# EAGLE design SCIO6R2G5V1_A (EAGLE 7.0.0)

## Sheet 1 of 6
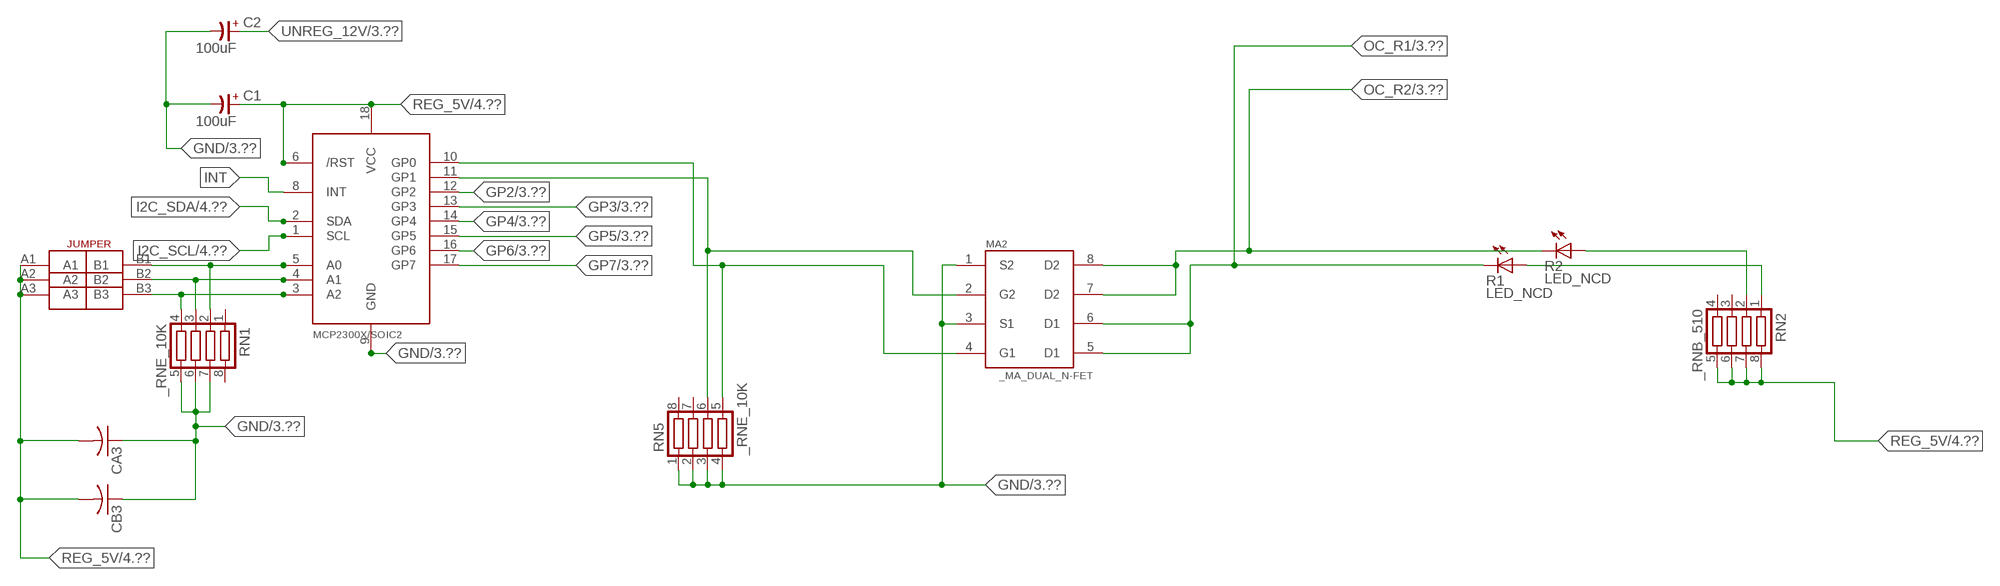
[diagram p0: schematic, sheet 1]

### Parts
C1  100uF  CP-E-025X060  [E-025X060]
C2  100uF  CP-E-025X060  [E-025X060]
CA3  CC1206KRX7R9BB104C1206K  [CC1206KRX7R9BB104]
CB3  TMK316F106ZL-TC1206K  [TMK316F106ZL-T]
IC2  MCP2300X/SO  [SO18W]
MA2  _MA_DUAL_N-FET  [_MA_DUAL_N-FET]
R1  LED_NCD  [CHIPLED_0603]
R2  LED_NCD  [CHIPLED_0603]
RN1  _RNE_10K  [RNE]
RN2  _RNB_510  [RNB]
RN5  _RNE_10K  [RNE]
U$18  JUMPER_3X2  [JUMPER_3X2]

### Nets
GND: C1.- C2.- CA3.1 CB3.1 IC2.9(GND) MA2.1(S2) MA2.3(S1) RN1.5 RN1.6 RN1.7 RN5.1 RN5.2 RN5.3 RN5.4 ; also sheet 3,4,6
GP2: IC2.12(GP2) ; also sheet 3
GP3: IC2.13(GP3) ; also sheet 3
GP4: IC2.14(GP4) ; also sheet 3
GP5: IC2.15(GP5) ; also sheet 3
GP6: IC2.16(GP6) ; also sheet 3
GP7: IC2.17(GP7) ; also sheet 3
I2C_SCL: IC2.1(SCL) ; also sheet 4
I2C_SDA: IC2.2(SDA) ; also sheet 4
INT: IC2.8(INT)
N$6: IC2.5(A0) RN1.2 U$18.B1
N$7: IC2.4(A1) RN1.3 U$18.B2
N$8: IC2.3(A2) RN1.4 U$18.B3
N$22: IC2.11(GP1) MA2.2(G2) RN5.6
N$23: IC2.10(GP0) MA2.4(G1) RN5.5
N$31: R2.A RN2.2
N$32: R1.A RN2.1
OC_R1: MA2.5(D1) MA2.6(D1) R1.C ; also sheet 3
OC_R2: MA2.7(D2) MA2.8(D2) R2.C ; also sheet 3
REG_5V: C1.+ CA3.2 CB3.2 IC2.6(/RST) IC2.18(VCC) RN2.5 RN2.6 RN2.7 RN2.8 U$18.A1 U$18.A2 U$18.A3 ; also sheet 4,6
UNREG_12V: C2.+ ; also sheet 3,4
Unconnected: RN1.1 RN1.8 RN2.3 RN2.4 RN5.7 RN5.8

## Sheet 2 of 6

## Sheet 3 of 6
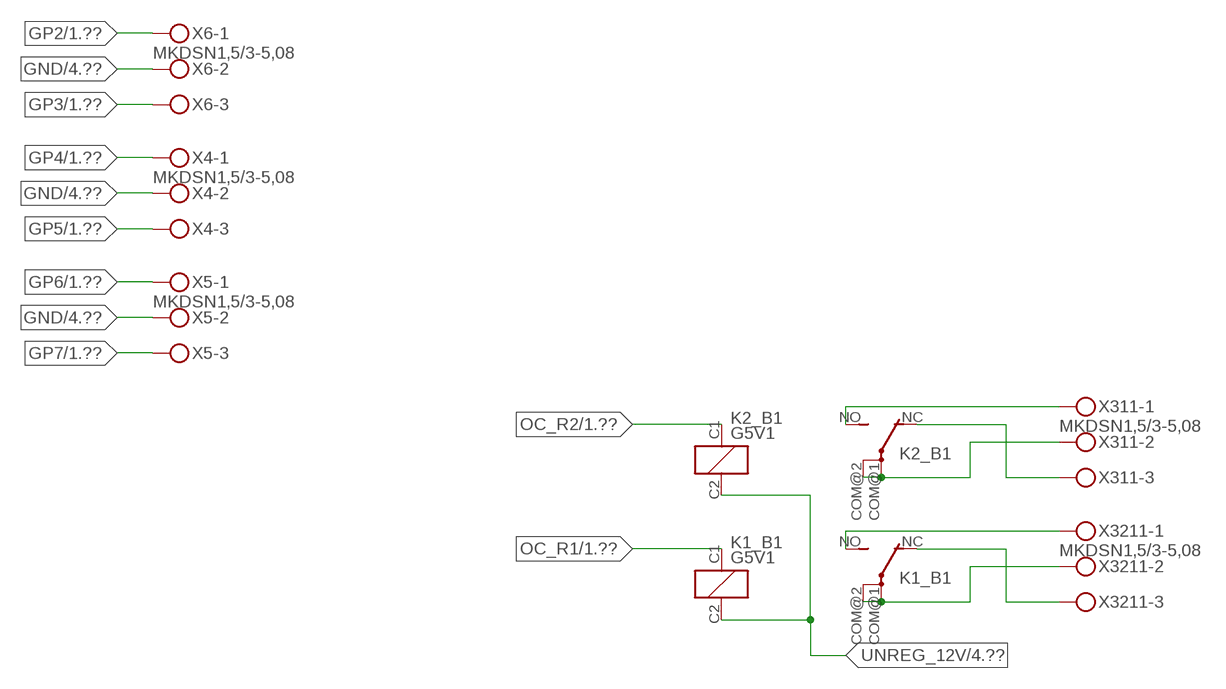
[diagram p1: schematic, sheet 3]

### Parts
K1_B1  G5V1  [G5V1]
K2_B1  G5V1  [G5V1]
X4  MKDSN1,5/3-5,08  [MKDSN1,5/3-5,08]
X5  MKDSN1,5/3-5,08  [MKDSN1,5/3-5,08]
X6  MKDSN1,5/3-5,08  [MKDSN1,5/3-5,08]
X311  MKDSN1,5/3-5,08  [MKDSN1,5/3-5,08]
X3211  MKDSN1,5/3-5,08  [MKDSN1,5/3-5,08]

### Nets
GND: X4.2 X5.2 X6.2 ; also sheet 1,4,6
GP2: X6.1 ; also sheet 1
GP3: X6.3 ; also sheet 1
GP4: X4.1 ; also sheet 1
GP5: X4.3 ; also sheet 1
GP6: X5.1 ; also sheet 1
GP7: X5.3 ; also sheet 1
N$221: K2_B1.NO(2:S) X311.1
N$222: K2_B1.NC(2:O) X311.3
N$223: K2_B1.COM@1(2:P) K2_B1.COM@2(2:P) X311.2
N$224: K1_B1.NO(2:S) X3211.1
N$225: K1_B1.NC(2:O) X3211.3
N$226: K1_B1.COM@1(2:P) K1_B1.COM@2(2:P) X3211.2
OC_R1: K1_B1.C1(1:C1) ; also sheet 1
OC_R2: K2_B1.C1(1:C1) ; also sheet 1
UNREG_12V: K1_B1.C2(1:C2) K2_B1.C2(1:C2) ; also sheet 1,4

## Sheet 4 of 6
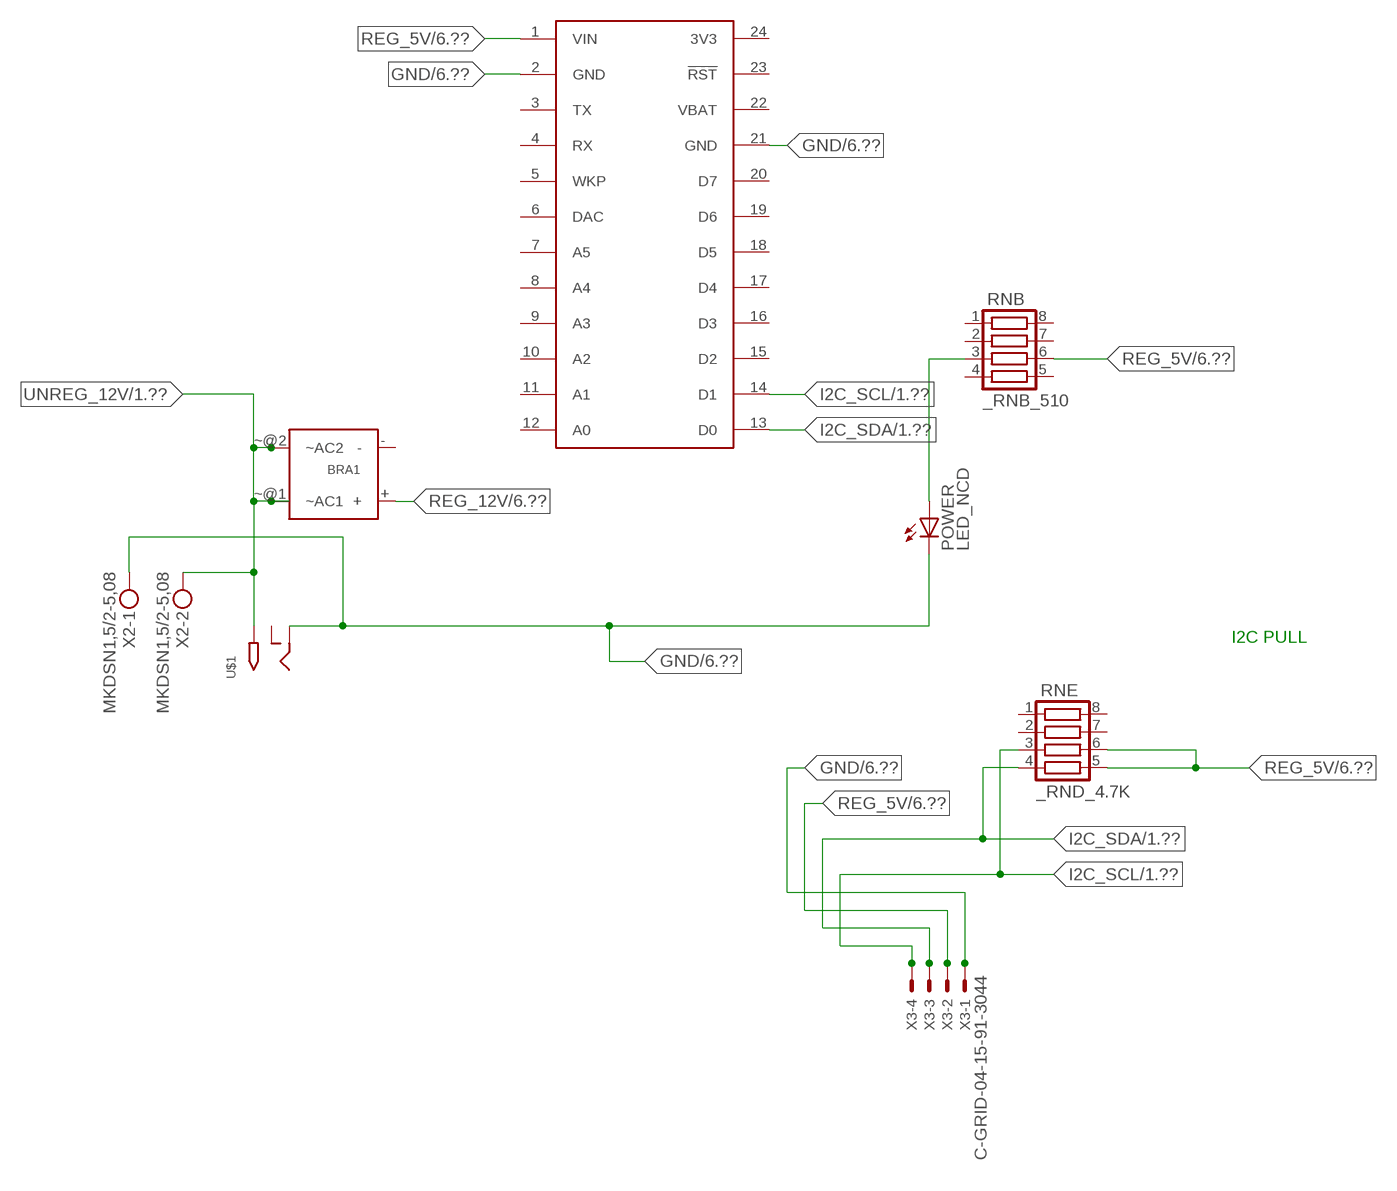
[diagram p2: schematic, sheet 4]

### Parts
BRA1  MB2S_  [MB2S]
POWER  LED_NCD  [CHIPLED_0603]
RNB  _RNB_510  [RNB]
RNE  _RND_4.7K  [RND]
S1  SPARK_CORECORE  [SPARK_CORE]
U$1  2.1MMJACK  [PJ-102A]
X2  MKDSN1,5/2-5,08  [MKDSN1,5/2-5,08]
X3  C-GRID-04-15-91-3044  [15-91-04]

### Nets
GND: POWER.C S1.2(GND) S1.21(GND) U$1.RING X2.1 X3.1 ; also sheet 1,3,6
I2C_SCL: RNE.3 S1.14(D1) X3.4 ; also sheet 1
I2C_SDA: RNE.4 S1.13(D0) X3.3 ; also sheet 1
N$2: POWER.A RNB.3
REG_5V: RNB.6 RNE.5 RNE.6 S1.1(VIN) X3.2 ; also sheet 1,6
REG_12V: BRA1.+ ; also sheet 6
UNREG_12V: BRA1.~@1(~AC1) BRA1.~@2(~AC2) U$1.TIP X2.2 ; also sheet 1,3
Unconnected: BRA1.- RNB.1 RNB.2 RNB.4 RNB.5 RNB.7 RNB.8 RNE.1 RNE.2 RNE.7 RNE.8 S1.3(TX) S1.4(RX) S1.5(WKP) S1.6(DAC) S1.7(A5) S1.8(A4) S1.9(A3) S1.10(A2) S1.11(A1) S1.12(A0) S1.15(D2) S1.16(D3) S1.17(D4) S1.18(D5) S1.19(D6) S1.20(D7) S1.23(!RST) U$1.RING_SW

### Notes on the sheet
- I2C PULL

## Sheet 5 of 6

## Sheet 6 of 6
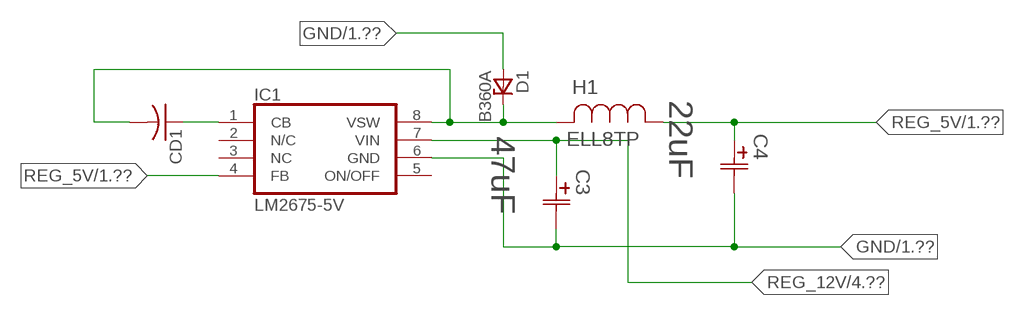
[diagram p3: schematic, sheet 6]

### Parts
C3  47uF  490-5463-6-NDCAP  [C2917(7343)-Y]
C4  22uF  490-5463-6-NDCAP  [C2917(7343)-Y]
CD1  _CD_10NF_50VC1206K  [_CD_10NF_50V]
D1  B360A  [DO214AC_ZENER]
H1  ELL8TP  [IND_ELL8TP]
IC1  LM2675-5V  LM2675  [SO-8]

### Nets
GND: C3.2(C2) C4.2(C2) D1.A IC1.6(GND) ; also sheet 1,3,4
N$1: CD1.2 D1.C H1.2 IC1.8(VSW)
N$3: CD1.1 IC1.1(CB)
REG_5V: C4.1(C1) H1.1 IC1.4(FB) ; also sheet 1,4
REG_12V: C3.1(C1) IC1.7(VIN) ; also sheet 4
Unconnected: IC1.2(N/C) IC1.5(ON/OFF)

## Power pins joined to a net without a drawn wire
3V3: S1.24(3V3)
NC: IC1.3(NC)
VBAT: S1.22(VBAT)

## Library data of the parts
BRA1 = NCD_ULTIMATE_LIBRARY:MB2S: Bridge Rectifier BRA MB2S 200V 500ma Digikey MB2S-TPMSTR-ND/MB2S-TP
C1 C2 = NCD_ULTIMATE_LIBRARY:CP-: Capacitors All Kinds POLARIZED CAP
C3 C4 = NCD_ULTIMATE_bhaskar:490-5463-6-ND: NCD CAP
CA3 = NCD_ULTIMATE_LIBRARY:CC1206KRX7R9BB104: Capacitor CA .1uF 50V SMT C1206K CC1206KRX7R9BB104
CB3 = NCD_ULTIMATE_LIBRARY:TMK316F106ZL-T: Capacitor CB 10uF SMT 1206 TMK316F106ZL-T
CD1 = NCD_ULTIMATE_LIBRARY:_CD_10NF_50V: Capacitor 10nF SMT
D1 = NCD_ULTIMATE_bhaskar:B360A: NCD DIODE B350A/B360A
H1 = NCD_ULTIMATE_bhaskar:ELL8TP: NCD coil
IC1 = NCD_ULTIMATE_bhaskar:LM2675: LM2675 NCD http://www.ti.com/lit/ds/symlink/lm2675.pdf
IC2 = NCD_ULTIMATE_LIBRARY:MCP2300X: Semiconductor Port Expander I/O 8-Bit I2C MCP23008 Inexpensive i2c i/o expander - 8 general purpose i/o pins with optional pullups
K1_B1 K2_B1 = NCD_ULTIMATE_LIBRARY:G5V1: RELAY 1 x switch, 0.5 A/125 V AC, 1 A/24 V DC , Omron
MA2 = NCD_ULTIMATE_LIBRARY:_MA_DUAL_N-FET: FET Dual N-Channel 8-SOIC NMOSFET Digikey 785-1064-2-ND/AO4842
POWER = NCD_ULTIMATE_bhaskar:LED_NCD
R1 R2 = NCD_ULTIMATE_LIBRARY:LED_NCD: LED Digikey 754-1132-2-ND/APT2012SRCPRV
RN1 RN5 = NCD_ULTIMATE_LIBRARY:_RNE_10K: Resistor Array RNE SMT 10K x 4 Single Resistor Source: http://www.ctscorp.com/components/Datasheets/CTSChipArrayDs.pdf Digikey 742C083103JPTR-ND/742C083103JP; OC_FARNELL: unknown; OC_NEWARK: unknown
RN2 RNB = NCD_ULTIMATE_LIBRARY:_RNB_510: Resistor Array RNB SMT 510 x 4 Single Resistor Source: http://www.ctscorp.com/components/Datasheets/CTSChipArrayDs.pdf Digikey 742C083511JPTR-ND/ 742C083511JP; OC_FARNELL: unknown; OC_NEWARK: unknown
RNE = NCD_ULTIMATE_LIBRARY:_RND_4.7K: Resistor Array RND SMT 4.7K x 4 Single Resistor Source: http://www.ctscorp.com/components/Datasheets/CTSChipArrayDs.pdf Digikey 742C083472JPTR-ND/742C083472JP; OC_FARNELL: unknown; OC_NEWARK: unknown
S1 = Spark:SPARK_CORE
U$1 = NCD_ULTIMATE_CONNECTORS:2.1MMJACK: 2.1mm x 5.5mm DC jack with internal switch. Digikey part #PJ-102A, 4UCON part #05537 By microbuilder.eu
U$18 = NCD_ULTIMATE_CONNECTORS:JUMPER_3X2
X2 = NCD_ULTIMATE_CONNECTORS:MKDSN1,5/2-5,08: MKDSN 1,5/ 2-5,08 Printklemme
X3 = NCD_ULTIMATE_CONNECTORS:C-GRID-04: CONNECTOR 4-Pos I2C wire to board 2.54 mm (0.100") pitch header Digikey WM1342-ND/0015912045; OC_FARNELL: unknown; OC_NEWARK: unknown
X4-X6 X311 X3211 = NCD_ULTIMATE_CONNECTORS:MKDSN1,5/3-5,08: MKDSN 1,5/ 3-5,08 Printklemme Nennstrom: 13,5 A Nennspannung: 250 V Rastermaß: 5,08 mm Polzahl: 3 Anschlussart: Schraubanschluss Montage: Löten Anschlussrichtung Leiter/Platine: 0 ° Artikelnummer: 1729131 Source: http://eshop.phoenixcontact.com .. 1729131.pdf

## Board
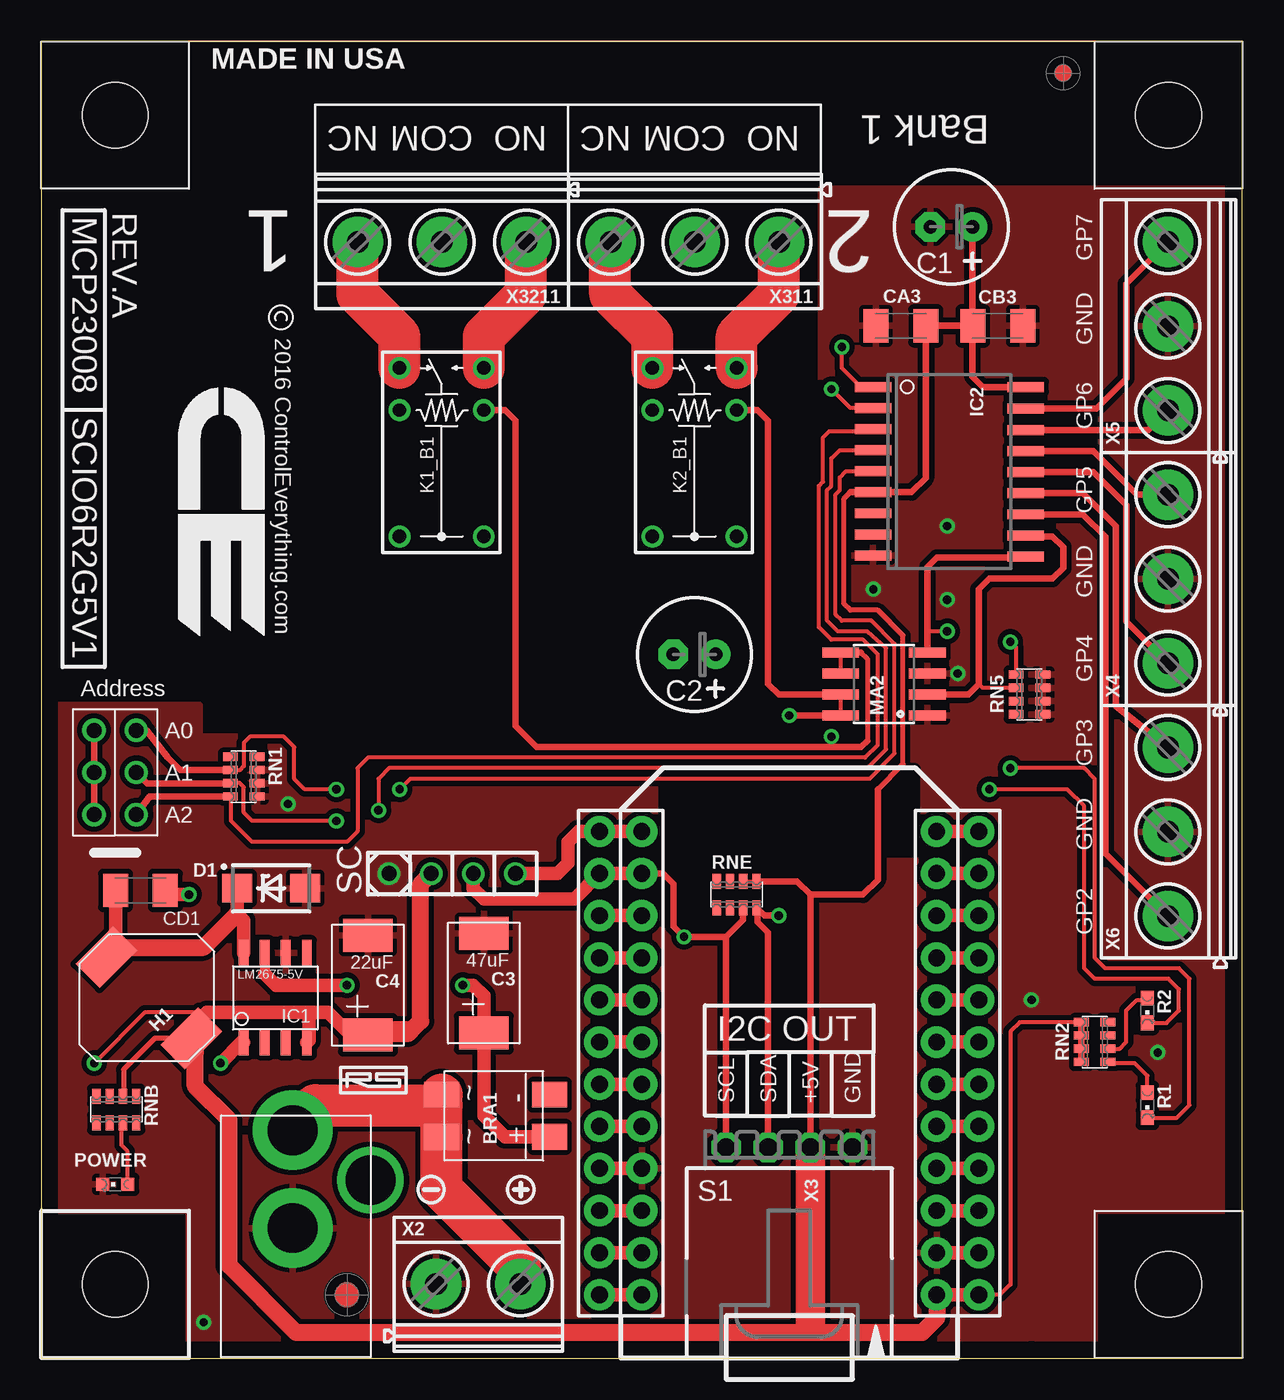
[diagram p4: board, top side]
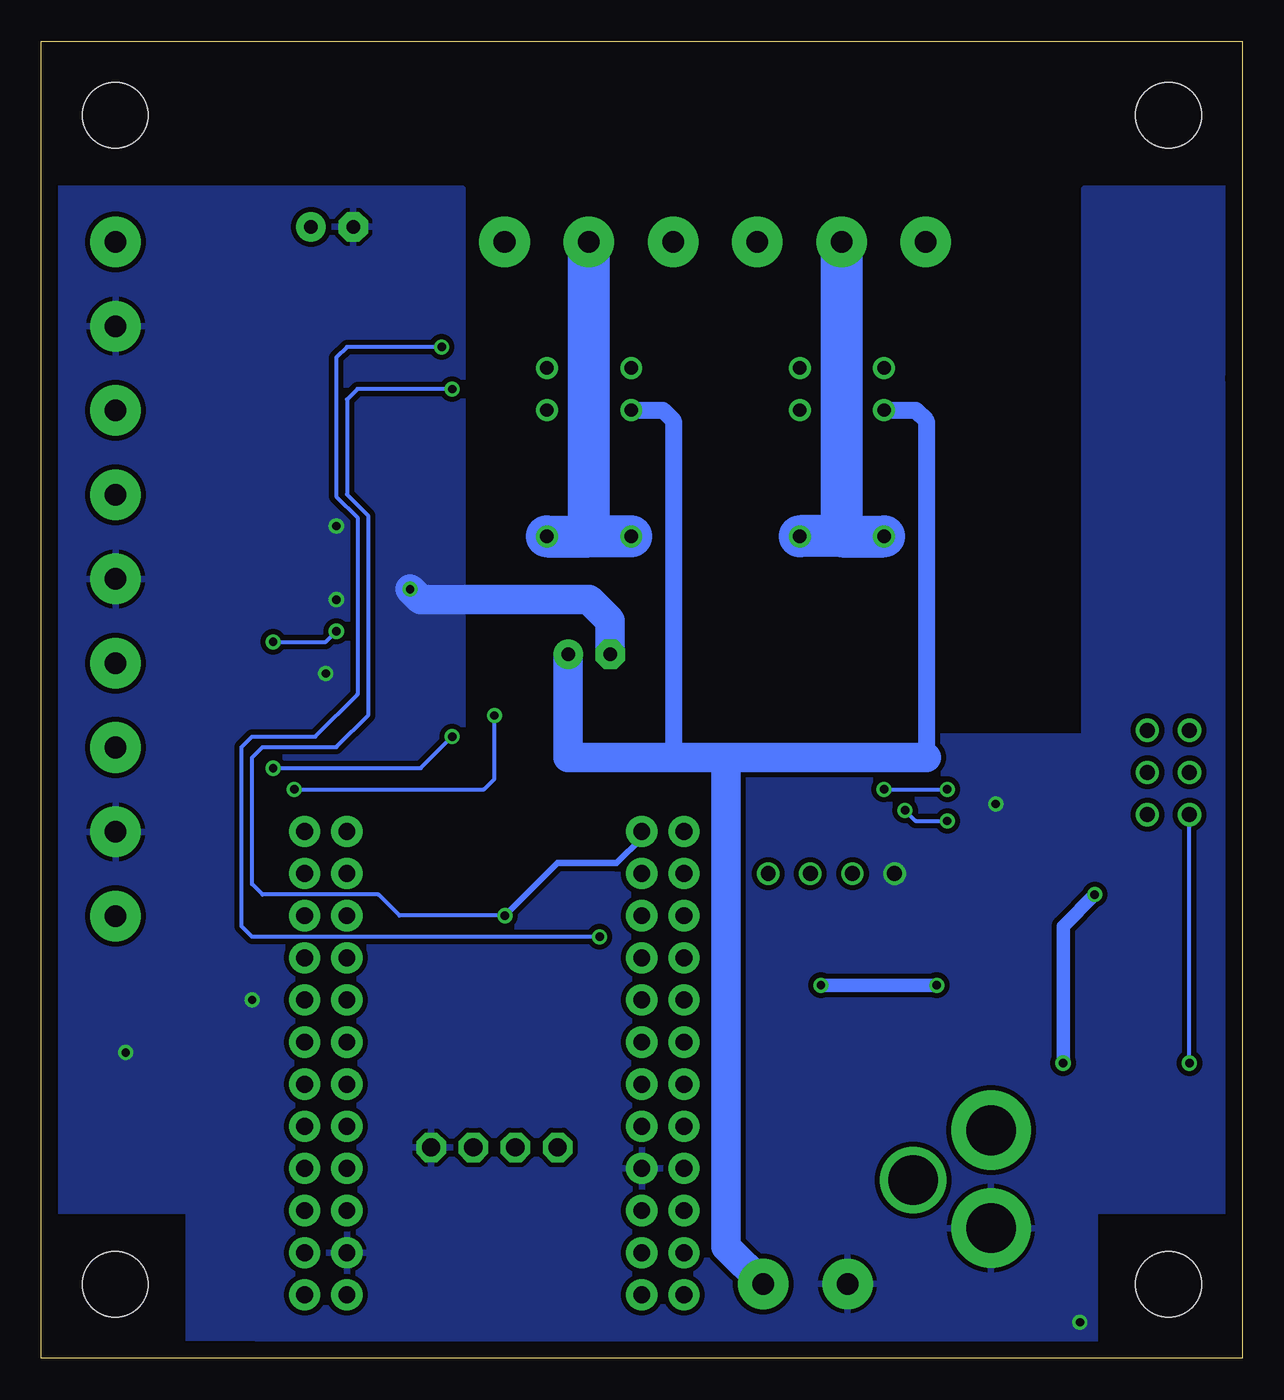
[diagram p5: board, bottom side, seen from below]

Size 72.39 x 79.38 mm. Coordinates in mm from the lower left corner, seen from the top.
Outline: 59.69,0 61.58,0
Outline: 0,59.99 0,59.05
Outline: 0,59.05 0,0 59.69,0
Outline: 59.69,0 72.39,0 72.39,79.38 0,79.38 0,59.05
Copper layers (1*16): Top 0.035mm / dielectric 1.5mm / Bottom 0.035mm
Design rules "default": minimum track width 10mil, minimum drill 24mil, track to track 8mil, track to pad 8mil, pad to pad 8mil, via to via 8mil, smd to smd 8mil, copper to edge 40mil, drill to drill 8mil, minimum pad ring 10mil, minimum via ring 8mil, stop-mask expansion 4mil, vias tented up to drill 0mil, thermal gap 10mil
Holes 3.96 mm at 4.45,4.45 4.45,4.45

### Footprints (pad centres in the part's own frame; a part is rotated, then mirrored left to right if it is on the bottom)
MB2S = smd 1.55 x 2.1: + 0,-6.5; - 2.54,-6.5; ~@1 0,0; ~@2 2.54,0
E-025X060 = drill 0.813 pad 1.778: + -1.27,0 | drill 0.813 pad 1.778 octagon: - 1.27,0
C2917(7343)-Y = smd 2 x 3: 1 -3,0; 2 3,0
CC1206KRX7R9BB104 = smd 1.5 x 2: 1 -1.5,0; 2 1.5,0
TMK316F106ZL-T = smd 1.5 x 2: 1 -1.5,0; 2 1.5,0
_CD_10NF_50V = smd 1.5 x 2: 1 -1.5,0; 2 1.5,0
DO214AC_ZENER = smd 1.8 x 1.7: A 2.05,0; C -2.05,0
IND_ELL8TP = smd 2.054 x 3.2 rotated 45: 1 -2.442,-2.696; 2 2.442,2.442
SO-8 = smd 0.6 x 1.55: 1 -1.905,-2.69; 2 -0.635,-2.69; 3 0.635,-2.69; 4 1.905,-2.69; 5 1.905,2.71; 6 0.635,2.71; 7 -0.635,2.71; 8 -1.905,2.71
SO18W = smd 0.6 x 2.2: 1 -4.445,-4.6; 2 -3.175,-4.6; 3 -1.905,-4.6; 4 -0.635,-4.6; 5 0.635,-4.6; 6 1.905,-4.6; 7 3.175,-4.6; 8 4.445,-4.6; 9 5.715,-4.6; 10 5.775,4.6; 11 4.505,4.6; 12 3.235,4.6; 13 1.965,4.6; 14 0.695,4.6; 15 -0.575,4.6; 16 -1.845,4.6; 17 -3.145,4.6; 18 -4.445,4.6
G5V1 = drill 0.813: C1 -2.54,2.54; C2 -2.54,-2.54; COM@1 5.08,-2.54; COM@2 5.08,2.54; NC -5.08,-2.54; NO -5.08,2.54
_MA_DUAL_N-FET = smd 0.61 x 2.21: 1 -1.905,-2.616; 2 -0.635,-2.616; 3 0.635,-2.616; 4 1.905,-2.616; 5 1.905,2.616; 6 0.635,2.616; 7 -0.635,2.616; 8 -1.905,2.616
CHIPLED_0603 = smd 0.8 x 0.8: A 0,-0.75; C 0,0.75
CHIPLED_0603' = smd 0.8 x 0.876: A 0,-0.75; C 0,0.75
RNE = smd 0.5 x 0.9: 1 -1.2,-0.8; 2 -0.4,-0.8; 3 0.4,-0.8; 4 1.2,-0.8; 5 1.2,0.8; 6 0.4,0.8; 7 -0.4,0.8; 8 -1.2,0.8
RNB = smd 0.5 x 0.9: 1 -1.2,-0.8; 2 -0.4,-0.8; 3 0.4,-0.8; 4 1.2,-0.8; 5 1.2,0.8; 6 0.4,0.8; 7 -0.4,0.8; 8 -1.2,0.8
RND = smd 0.5 x 0.9: 1 -1.2,-0.8; 2 -0.4,-0.8; 3 0.4,-0.8; 4 1.2,-0.8; 5 1.2,0.8; 6 0.4,0.8; 7 -0.4,0.8; 8 -1.2,0.8
SPARK_CORE = drill 1.016 pad 1.88: 1 -8.89,13.97; 2 -8.89,11.43; 3 -8.89,8.89; 4 -8.89,6.35; 5 -8.89,3.81; 6 -8.89,1.27; 7 -8.89,-1.27; 8 -8.89,-3.81; 9 -8.89,-6.35; 10 -8.89,-8.89; 11 -8.89,-11.43; 12 -8.89,-13.97; 13 8.89,-13.97; 14 8.89,-11.43; 15 8.89,-8.89; 16 8.89,-6.35; 17 8.89,-3.81; 18 8.89,-1.27; 19 8.89,1.27; 20 8.89,3.81; 21 8.89,6.35; 22 8.89,8.89; 23 8.89,11.43; 24 8.89,13.97; 25 -11.43,13.97; 26 -11.43,11.43; 27 -11.43,8.89; 28 -11.43,6.35; 29 -11.43,3.81; 30 -11.43,1.27; 31 -11.43,-1.27; 32 -11.43,-3.81; 33 -11.43,-6.35; 34 -11.43,-8.89; 35 -11.43,-11.43; 36 -11.43,-13.97; 37 11.43,13.97; 38 11.43,11.43; 39 11.43,8.89; 40 11.43,6.35; 41 11.43,3.81; 42 11.43,1.27; 43 11.43,-1.27; 44 11.43,-3.81; 45 11.43,-6.35; 46 11.43,-8.89; 47 11.43,-11.43; 48 11.43,-13.97
PJ-102A = drill 3 pad 4.8: RING 0.1,-3.39; TIP 0.1,-9.29 | drill 3 pad 3.251: RING_SW -4.6,-6.29
PCB_MOUNTING_HOLE = hole 3.962: 4.445,4.445
JUMPER_3X2 = drill 0.9: A1 0,5.08; A2 0,2.54; A3 0,0; B1 2.54,5.08; B2 2.54,2.54; B3 2.54,0
MKDSN1,5/2-5,08 = drill 1.3 pad 3.048: 1 -2.561,0.025; 2 2.519,0.025
15-91-04 = drill 1.1 pad 1.778 octagon: 1 -3.81,-7.62; 2 -1.27,-7.62; 3 1.27,-7.62; 4 3.81,-7.62
MKDSN1,5/3-5,08 = drill 1.3 pad 3.048: 1 -7.641,0.025; 2 -2.561,0.025; 3 2.519,0.025

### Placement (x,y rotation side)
BRA1  24.13,13.34 90 top
C1  54.86,68.2 180 top
C2  39.37,42.42 180 top
C3  26.67,22.61 90 top
C4  19.68,22.48 90 top
CA3  51.82,62.23 0 top
CB3  57.66,62.23 180 top
CD1  5.97,28.19 180 top
D1  13.84,28.32 0 top
H1  6.35,21.72 90 top
IC1  14.1,21.72 0 top
IC2  54.74,54.1 270 top
K1_B1  24.13,54.61 270 top
K2_B1  39.37,54.61 270 top
MA2  50.8,40.64 90 top
POWER  4.45,10.48 90 top
R1  LED_NCD  [CHIPLED_0603']  66.67,15.24 180 top
R2  LED_NCD  [CHIPLED_0603']  66.67,20.96 180 top
RN1  12.19,35.05 270 top
RN2  63.5,19.05 90 top
RN5  59.56,40 90 top
RNB  4.51,14.99 0 top
RNE  41.91,27.94 0 top
S1  45.09,17.78 180 top
U$1  15.24,4.45 180 top
U$4  PCB_MOUNTING_HOLE  [PCB_MOUNTING_HOLE]  72.39,70.48 90 top
U$6  PCB_MOUNTING_HOLE  [PCB_MOUNTING_HOLE]  72.39,0 90 top
U$10  [VISION_REF15]  18.41,3.81 0 top
U$11  PCB_MOUNTING_HOLE  [PCB_MOUNTING_HOLE]  8.89,70.48 90 top
U$18  3.17,32.77 0 top
U$19  [VISION_REF10]  61.59,77.47 0 top
U$21  [ICON_USA]  21.97,78.99 180 top
U$22  [ICON_MINUS]  23.5,10.16 180 top
U$24  [ICON_PLUS]  28.89,10.16 90 top
X2  26.35,4.45 0 top
X3  45.09,5.08 180 top
X4  67.94,49.53 90 top
X5  67.94,64.77 90 top
X6  67.94,34.29 90 top
X311  36.83,67.31 180 top
X3211  21.59,67.31 180 top

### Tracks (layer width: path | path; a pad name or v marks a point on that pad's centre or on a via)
GND  (via drill 0.5, 0.9)
  Bottom 1.778: C2.- 38.1,44.45 39.37,45.72 49.53,45.72 v50.16,46.35
  other vias: 14.86,33.4 54.61,45.72 54.61,50.16 59.69,21.59 67.31,18.41 55.24,41.27 9.78,2.16 20.95,29.21
  pour Bottom (isolate 0.305): -3.81,8.89 8.89,8.89 8.89,0 63.5,0 63.5,8.89 71.75,8.89 71.75,70.48 46.99,70.48 46.99,37.46 9.53,37.46 9.53,70.48 -3.81,70.48
  pour Top (isolate 0.305): -8.26,8.89 8.89,8.89 8.89,0 63.5,0 63.5,8.89 71.75,8.89 71.75,70.48 46.99,70.48 46.99,37.46 9.53,37.46 9.53,39.37 -8.26,39.37
GP2
  Top 0.406: IC2.12 62.8,50.87 64.14,49.53 64.14,30.43 X6.1
GP3
  Top 0.406: IC2.13 62.8,52.14 64.77,50.16 64.77,39.32 X6.3
GP4
  Top 0.406: IC2.14 63.43,53.41 65.41,51.43 65.41,44.4 X4.1
GP5
  Top 0.406: IC2.15 63.43,54.68 66.04,52.07 67.9,52.07 X4.3
GP6
  Top 0.406: IC2.16 66.74,55.95 X5.1
GP7
  Top 0.406: IC2.17 63.6,57.25 65.41,59.05 65.41,64.77 X5.3
I2C_SCL  (via drill 0.5, 0.9)
  Top 0.254: IC2.1 49.4,58.55 48.26,59.69 v48.26,60.96
  Top 0.406: X3.4 41.27,25.4 | 41.27,25.4 42.29,26.42 42.29,27.12 RNE.3 | S1.14 37.47,29.21 38.1,28.57 38.1,26.04 v38.73,25.4 41.27,25.4
  Top 0.813: v26.04,29.21 26.04,28.32 26.67,27.69 32.13,27.69 33.66,29.21
  Bottom 0.254: v48.26,60.96 53.98,60.96 54.61,60.32 54.61,51.94 53.34,50.67 53.34,40 55.88,37.46 59.69,37.46 60.33,36.83 60.33,26.04 59.69,25.4 v38.73,25.4
I2C_SDA  (via drill 0.5, 0.9)
  Top 0.254: IC2.2 48.77,57.28 v47.62,58.42
  Top 0.406: X3.3 43.81,25.65 43.18,26.29 43.18,27.07 RNE.4 43.58,26.67 v44.45,26.67
  Top 0.813: v28.57,29.21 31.11,29.21 31.75,29.85 31.75,31.12 32.38,31.75 33.66,31.75
  Bottom 0.254: v47.62,58.42 53.34,58.42 53.98,57.78 53.98,52.07 52.7,50.8 52.7,38.73 54.61,36.83 59.05,36.83 59.69,36.2 59.69,28.57 59.05,27.94 52.07,27.94 50.8,26.67 v44.45,26.67
  Bottom 0.406: S1.13 36.2,31.37 37.72,29.85 41.27,29.85 v44.45,26.67
N$1
  Top 0.813: H1.2 3.88,24.77 | D1.C 11.79,26.78 12.19,26.38 IC1.8 | CD1.2 4.47,24.79 4.45,24.77
  Top 1.016: 3.88,24.77 4.45,24.77 9.78,24.77 11.79,26.78
N$2
  Top 0.254: POWER.A 5.2,12.46 4.83,12.83 4.83,14.1 RNB.3
  Top 0.406: 4.95,14.14 RNB.3
N$3  (via drill 0.5)
  Top 0.813: IC1.1 12.04,19.03 v10.79,17.78 | v8.89,27.94 7.72,27.94 CD1.1
  Bottom 0.813: v10.79,17.78 10.79,26.04 v8.89,27.94
N$6  (via drill 0.5)
  Top 0.254: v21.59,34.29 22.23,34.92 49.91,34.92 51.44,36.45 51.44,43.05 50.04,44.45 48.26,44.45 47.88,44.83 47.88,52.07 48.13,52.32 48.13,53.09 48.51,53.47 IC2.5 50.01,53.34 | v17.78,34.29 15.88,34.29 15.24,34.92 15.24,36.83 14.61,37.46 12.57,37.46 12.19,37.08 12.19,35.69 11.94,35.43 11.41,35.43 RN1.2
  Top 0.406: RN1.2 8.36,35.45 7.62,36.2 6.35,37.85 U$18.B1
  Bottom 0.254: v21.59,34.29 v17.78,34.29
N$7  (via drill 0.5)
  Top 0.254: v20.32,33.02 20.32,34.92 20.95,35.56 49.78,35.56 50.93,36.7 50.93,42.8 49.78,43.81 48.01,43.81 47.37,44.45 47.37,52.32 47.62,52.58 47.62,54.23 48.13,54.74 IC2.4 50.01,54.61 | v17.78,32.38 12.7,32.38 12.19,32.89 12.19,34.42 11.94,34.67 11.41,34.67 RN1.3
  Top 0.406: RN1.3 6.37,34.65 U$18.B2
  Bottom 0.254: v20.32,33.02 19.68,32.38 v17.78,32.38
N$8
  Top 0.254: RN1.4 11.43,33.81 11.43,32.38 12.7,31.12 18.41,31.12 19.05,31.75 19.05,35.56 19.68,36.2 49.66,36.2 50.42,36.96 50.42,42.42 49.53,43.31 47.62,43.31 46.86,44.07 46.86,52.58 47.12,52.83 47.12,55.5 47.5,55.88 50.01,55.88 IC2.3
  Top 0.406: RN1.4 6.53,33.85 U$18.B3
N$22
  Top 0.254: RN5.6 56.75,40.4 56.52,40.64
  Top 0.406: MA2.2 55.88,40 56.52,40.64 56.52,46.35 57.15,46.99 60.96,46.99 61.59,47.62 61.59,48.89 60.96,49.53 59.4,49.53 IC2.11
N$23  (via drill 0.5)
  Top 0.254: RN5.5 58.76,42.84 v58.42,43.18 | v54.61,43.81 53.42,43.81
  Top 0.406: MA2.4 53.42,43.81 53.42,47.7 53.98,48.26 59.27,48.26 IC2.10
  Bottom 0.254: v58.42,43.18 55.24,43.18 v54.61,43.81
N$31
  Top 0.254: RN2.2 65,18.65 65.41,19.05 65.41,20.96 66.04,21.59 66.56,21.59 R2.A
N$32
  Top 0.254: R1.A 66.67,17.02 65.91,17.78 64.37,17.78 RN2.1
N$221
  Top 2.54: K2_B1.NO 41.91,61.59 44.45,64.14 44.45,67.26 X311.1
N$222
  Top 2.54: K2_B1.NC 36.83,61.59 34.29,64.14 34.29,67.26 X311.3
N$223
  Bottom 2.54: K2_B1.COM@1 39.37,49.53 | K2_B1.COM@2 39.37,49.53 | 39.37,49.53 39.37,67.26 X311.2
N$224
  Top 2.54: K1_B1.NO 26.67,61.59 29.21,64.14 29.21,67.26 X3211.1
N$225
  Top 2.54: K1_B1.NC 21.59,61.59 19.05,64.14 19.05,67.26 X3211.3
N$226
  Bottom 2.54: X3211.2 24.15,49.55 | 24.15,49.55 24.13,49.53 K1_B1.COM@1 | 24.15,49.55 26.65,49.55 K1_B1.COM@2
OC_R1  (via drill 0.5)
  Top 0.254: MA2.5 MA2.6 | R1.C 68.47,14.49 69.22,15.24 69.22,22.86 68.58,23.5 64.14,23.5 63.5,24.13 63.5,34.92 62.87,35.56 v58.42,35.56 | v47.62,37.46 47.62,36.83
  Top 0.305: 49.4,42.54 49.78,42.16 49.78,37.21
  Top 0.406: MA2.5 49.4,42.54 | 49.78,37.21 49.4,36.83 47.62,36.83 29.84,36.83 28.57,38.1 28.57,56.52 27.94,57.15 K1_B1.C1
  Bottom 0.254: v58.42,35.56 49.53,35.56 v47.62,37.46
OC_R2  (via drill 0.5)
  Top 0.254: MA2.7 MA2.8 | R2.C 67.83,20.21 68.58,20.96 68.58,22.23 67.94,22.86 63.5,22.86 62.87,23.5 62.87,33.27 61.85,34.29 v57.15,34.29
  Top 0.406: K2_B1.C1 43.18,57.15 43.81,56.52 43.81,40.64 44.45,40 MA2.7 | MA2.8 v45.09,38.73
  Bottom 0.254: v57.15,34.29 45.72,34.29 45.09,34.92 v45.09,38.73
REG_5V  (via drill 0.5, 0.9)
  Top 0.254: RN2.5 58.98,20.25 58.42,19.69 58.42,4.45 57.78,3.81 56.52,3.81 | RNE.6 RNE.5 | 9.96,20.83 6.22,20.83 v3.17,17.78
  Top 0.305: 50.42,34.29 51.94,35.81 51.94,43.56 50.42,45.08 48.77,45.08 48.39,45.47 48.39,51.82 48.77,52.2 | H1.1 6.83,19.28 4.95,17.4 4.95,15.83 RNB.6
  Top 0.406: U$18.A3 U$18.A2 U$18.A1 | RN2.8 RN2.7 RN2.6 RN2.5 | 48.77,52.2 IC2.6 52.45,52.2 53.32,53.06 CA3.2 CB3.2 56.13,62.21 | IC2.18 56.77,58.55 56.13,59.18 56.13,62.21 | C1.+ 56.13,62.21 | RNE.5 45.55,28.74 46.35,27.94 | 46.35,27.94 X3.2 | 50.42,34.29 50.42,28.83 49.53,27.94 46.35,27.94
  Top 0.813: 16.13,20.83 9.96,20.83 H1.1 | 16.13,20.83 17.27,20.83 18.41,19.69 20.75,19.69 C4.1 | IC1.4 16.13,19.15 16.13,20.83
  Top 1.016: 46.35,2.16 46.35,1.52 | 46.35,1.52 15.37,1.52 11.3,5.59 11.3,14.35 9.27,16.38 9.27,18.41 H1.1 | 22.05,19.69 22.23,19.69 22.86,20.32 22.86,28.57 v23.5,29.21 | S1.1 53.98,2.41 53.09,1.52 46.35,1.52
  Top 1.27: 20.75,19.69 22.05,19.69
  Top 1.778: X3.2 46.35,2.16
  Bottom 0.254: v3.17,17.78 U$18.A3
REG_12V  (via drill 0.5)
  Top 0.61: IC1.7 13.46,23.16 | 14.1,22.48 14.15,22.48
  Top 0.813: v18.41,22.48 14.15,22.48 13.46,23.16 | v25.4,22.48 26.04,22.48 26.67,21.84 C3.1 26.67,14.61 27.94,13.34 BRA1.+
  Bottom 0.813: v18.41,22.48 v25.4,22.48
UNREG_12V
  Top 2.54: X2.2 28.87,5.42 24.13,10.16 BRA1.~@1 24.13,15.24 | 24.13,15.24 BRA1.~@2 | U$1.TIP 15.14,13.87 16.51,15.24 24.13,15.24
  Bottom 1.016: K1_B1.C2 19.68,57.15 19.05,56.52 19.05,36.2 | K2_B1.C2 34.92,57.15 34.29,56.52 34.29,36.83 33.66,36.2
  Bottom 1.778: 31.11,36.2 33.66,36.2 40.64,36.2 C2.+ | 31.11,36.2 19.05,36.2 | 31.11,36.2 31.11,6.71 X2.2

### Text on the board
tNames: Bank 1 | NC | COM | NO | NC | COM | NO | MCP23008 | REV.A | 1 | 2 | GP7 | 2016 ControlEverything.com | GND | SCIO6R2G5V1 | GP6 | GP5 | GND | GP4 | Address | A0 | GP3 | A1 | A2 | GND | SC | GP2 | I2C OUT | SCL | SDA | +5V | GND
